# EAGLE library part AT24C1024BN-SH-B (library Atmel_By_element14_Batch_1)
Two-wire Serial EEPROM
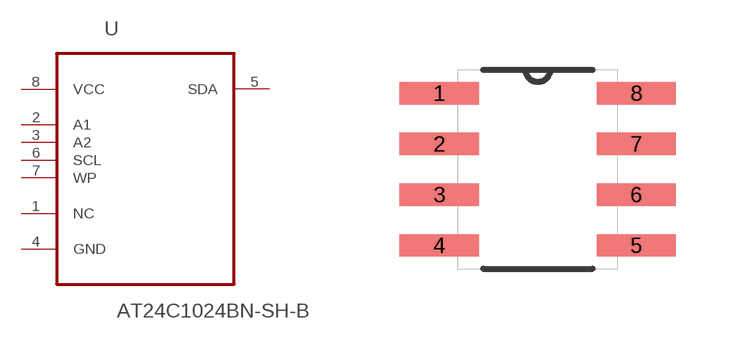
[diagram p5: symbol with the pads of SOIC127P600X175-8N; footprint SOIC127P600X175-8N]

Designator prefix U

## AT24C1024BN-SH-B (MPN: AT24C1024BN-SH-B; OC_FARNELL: 1636610; OC_NEWARK: 03P2043; PACKAGE: SOIC-8; SUPPLIER: Atmel)  [SOIC127P600X175-8N]
1  NC  nc
2  A1  in
3  A2  in
4  GND  pas
5  SDA
6  SCL  in
7  WP  in
8  VCC  pwr

## Footprint SOIC127P600X175-8N (pad centres in mm)
smd 1.981 x 0.559: 1 -2.464,1.905; 2 -2.464,0.635; 3 -2.464,-0.635; 4 -2.464,-1.905; 5 2.464,-1.905; 6 2.464,-0.635; 7 2.464,0.635; 8 2.464,1.905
